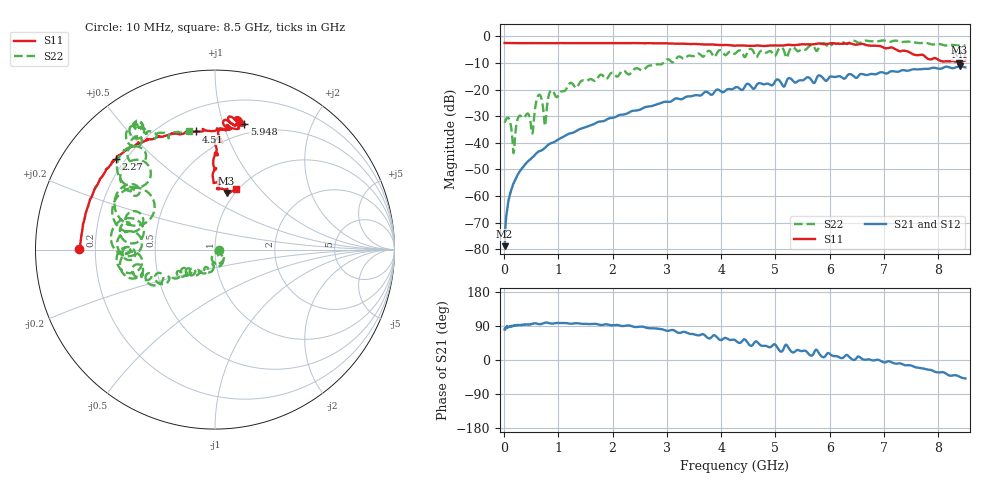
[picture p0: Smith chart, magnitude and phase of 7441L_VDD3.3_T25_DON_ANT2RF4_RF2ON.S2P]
!Agilent Technologies,E5071C,MY46417908,A.11.23
!Date: Mon May 03 19:54:09 2021
!Data & Calibration Information:
!Freq	S11:SOLT2(ON)	S21:SOLT2(ON)	S12:SOLT2(ON)	S22:SOLT2(ON)
!PortZ  Port1:50+j0  Port2:50+j0
!Above PortZ is port z conversion or system Z0 setting when saving the data.
!When reading, reference impedance value at option line is always used.
# Hz S dB R 50
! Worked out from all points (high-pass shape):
!   1601 points, 10 MHz to 8.5 GHz, reference 50 ohm
!   highest |S21| = -11.25 dB at 8.399 GHz (marker M1); lowest = -78.9 dB at 10 MHz (marker M2)
!   |S21| within 3 dB of the highest: 6.732 GHz to 6.814 GHz (81.86 MHz wide, 1.21 % of centre); 6.849 GHz to end of sweep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
!   lowest |S11| = -9.9 dB at 8.389 GHz (marker M3), VSWR 1.95, Z = 46 + j32.3 ohm
!   |S11| at or under -10 dB: nowhere
!   |S22| runs from -43.9 to -1.5 dB; largest |S21 - S12| = 0.0019
!   S11 on the Smith chart (normalised r, x): 10 MHz: 0.14, +0.00; 2.27 GHz: 0.16, +0.38; 4.51 GHz: 0.34, +0.79; 5.948 GHz: 0.40, +1.18; 8.5 GHz: 0.97, +0.75
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1e7  -2.44 179.7  -78.85 80.5  -78.28 65.6  -32.45 0.3
7.898125e7  -2.48 178.2  -62.18 87.3  -62.01 88.6  -30.61 -33.3
1.798e8  -2.51 176.0  -55.11 91.4  -55.06 91.0  -43.67 -17.3
3.124562e8  -2.53 173.3  -50.09 91.8  -50.08 92.2  -29.94 -43.5
5.140938e8  -2.52 169.1  -45.67 95.3  -45.67 95.6  -36.11 -63.7
6.361375e8  -2.53 166.4  -43.29 94.7  -43.27 94.8  -22.03 -63.8
7.52875e8  -2.52 164.2  -41.95 98.3  -41.92 98.1  -33.66 -80.0
8.643062e8  -2.53 162.0  -40.15 96.1  -40.13 96.3  -20.27 -76.8
1.426769e9  -2.51 151.7  -34.59 95.6  -34.60 95.6  -16.67 -114.8
2.270462e9  -2.51 137.5  -28.93 91.1  -28.94 91.2  -14.02 -149.1
2.843538e9  -2.61 130.4  -25.38 82.4  -25.39 82.4  -10.47 -149.9
4.255e9  -3.48 105.3  -19.22 52.6  -19.22 52.6  -6.49 -178.5
4.5097e9  -3.52 99.2  -17.92 41.3  -17.92 41.2  -5.05 179.8
5.088081e9  -3.46 85.0  -16.95 23.2  -16.92 23.2  -4.22 158.2
5.210125e9  -3.21 83.5  -16.56 39.1  -16.56 38.9  -7.98 154.4
5.295025e9  -3.27 83.4  -16.07 21.9  -16.06 22.0  -4.19 155.2
5.671769e9  -2.99 77.3  -16.73 11.6  -16.68 11.5  -3.27 135.8
5.947694e9  -2.84 76.9  -16.59 16.1  -16.58 16.3  -3.47 125.6
7.088538e9  -4.33 87.7  -13.53 -3.0  -13.56 -3.0  -2.01 121.1
8.388569e9  -9.85 78.5  -11.26 -43.8  -11.29 -43.8  -3.47 105.0
8.399181e9  -9.83 77.5  -11.25 -44.7  -11.29 -44.7  -3.47 104.7
8.5e9  -8.96 71.0  -11.63 -48.7  -11.65 -48.8  -3.39 102.1
